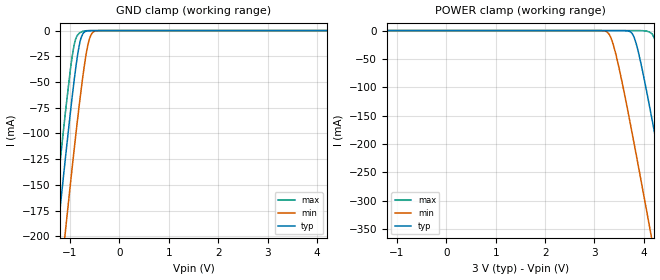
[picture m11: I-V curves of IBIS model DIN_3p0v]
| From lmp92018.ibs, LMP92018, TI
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|   Model
[Model]   DIN_3p0v
Model_type   Input
Vinl = 0.9
Vinh = 2.1
|   typ   min   max
C_comp   0.3672pF   0.3049pF   0.3707pF
[Voltage Range]   3   2.7   3.3
[Temperature Range]   27   125   -40
[Power Clamp Reference]   3   2.7   3.3
[GND Clamp Reference]   0   0   0
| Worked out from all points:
|   GND clamp passes 1 mA (typ) near -0.69 V on its own axis
[GND Clamp]
|   Voltage   I(typ)   I(min)   I(max)
-3V       -1.048A    -1.117A    -1.005A
-1.353V   -244.5mA   -316.3mA   -199.1mA
-1.335V   -236mA     -307.8mA   -190.6mA
-1.191V   -168.5mA   -240.1mA   -123.3mA
-1.083V   -119.2mA   -190.2mA   -74.92mA
-921mV    -50.14mA   -117.7mA   -15mA
-849mV    -24.41mA   -86.98mA   -4.465mA
-777mV    -7.153mA   -58.11mA   -1.447mA
-687mV    -833.5uA   -26.81mA   -207.4uA
-615mV    -139.1uA   -9.433mA   -26.54uA
-471mV    -2.731uA   -289.3uA   0A
5.991V    0A         0A         0A
[POWER Clamp]
|   Voltage   I(typ)   I(min)   I(max)
-3V       0A         0A         0A
3.237V    0A         -1.661mA   0A
3.417V    -534.6nA   -36.39mA   0A
3.777V    -7.144mA   -187.5mA   0A
3.885V    -36.58mA   -237.3mA   -10.04uA
4.101V    -127.3mA   -339.1mA   -2.139mA
4.155V    -151.9mA   -364.8mA   -4.899mA
4.263V    -202mA     -416.5mA   -27.31mA
4.533V    -330.4mA   -546.7mA   -142.7mA
4.875V    -496mA     -713.1mA   -305.5mA
5.271V    -689.7mA   -906.8mA   -498.4mA
5.991V    -1.044A    -1.259A    -852.8mA
